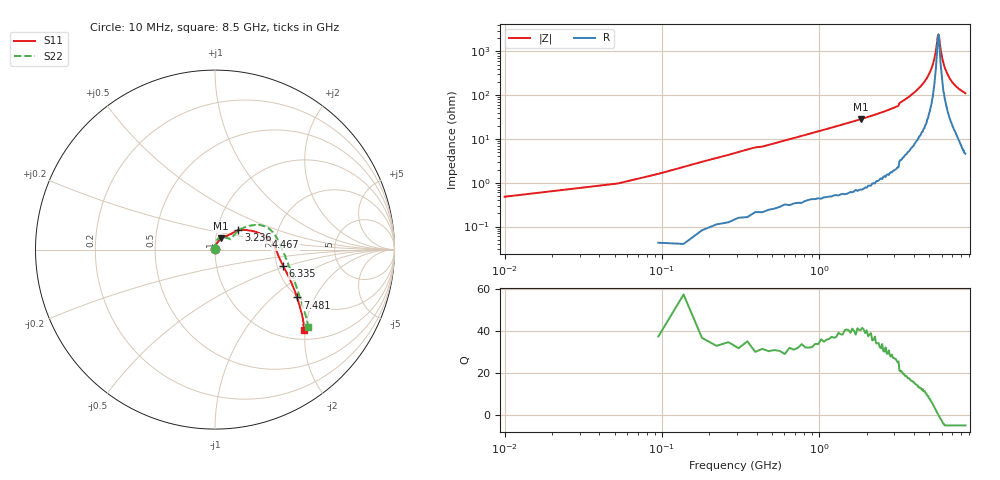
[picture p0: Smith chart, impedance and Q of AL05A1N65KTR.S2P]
!AVX Corporation
!PN: AL05A1N65KTR
!Description: Air Core Inductor, 1.65nH, 2 Turns
!Agilent Technologies,E5071C,MY46102230,A.09.54
!Date: Mon Sep 03 16:13:00 2012
!Data & Calibration Information:
!Freq	S11:SOLT2(ON)	S21:SOLT2(ON)	S12:SOLT2(ON)	S22:SOLT2(ON)
# Hz S dB R 50
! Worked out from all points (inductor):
!   201 points, 10 MHz to 8.5 GHz, reference 50 ohm
!   read as 1/Y11, port 2 shorted: L = 2.67 nH near 52.45 MHz
!   highest Q = 40.6 at 1.835 GHz (marker M1), where L = 2.45 nH
!   self-resonance near 5.728 GHz
!   S11 on the Smith chart (normalised r, x): 10 MHz: 1.00, +0.00; 3.236 GHz: 1.26, +0.28; 4.467 GHz: 1.77, +0.27; 6.335 GHz: 2.16, -0.46; 7.481 GHz: 1.97, -1.46; 8.5 GHz: 1.21, -1.96
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1e7  -58.61 74.1  -0.01 -0.2  -0.10 -0.5  -55.87 62.4
5.245e7  -46.79 83.3  -0.00 -0.8  0.02 -0.9  -46.65 84.5
9.49e7  -42.16 82.5  -0.01 -1.4  0.01 -1.4  -42.47 82.3
1.798e8  -36.85 81.4  -0.01 -2.6  0.00 -2.6  -36.81 82.9
3.496e8  -31.48 78.3  -0.02 -5.0  -0.01 -5.1  -31.54 83.5
3.9205e8  -30.72 78.7  -0.03 -5.6  -0.02 -5.7  -30.74 81.9
4.345e8  -31.84 76.9  -0.03 -6.1  -0.01 -6.2  -31.84 81.7
6.043e8  -29.25 74.1  -0.04 -8.5  -0.03 -8.6  -29.33 79.4
9.0145e8  -26.52 71.2  -0.06 -12.6  -0.05 -12.7  -26.63 77.0
1.4533e9  -24.07 65.9  -0.10 -20.4  -0.10 -20.4  -24.07 72.9
1.83535e9  -22.92 62.6  -0.13 -25.8  -0.13 -25.8  -22.90 67.8
2.85415e9  -20.60 52.3  -0.18 -40.4  -0.18 -40.5  -20.43 42.8
3.19375e9  -19.78 48.6  -0.20 -45.5  -0.19 -45.6  -19.67 33.5
3.2362e9  -15.45 39.9  -0.29 -46.7  -0.29 -46.7  -15.18 40.0
3.70315e9  -13.10 28.6  -0.40 -54.0  -0.40 -54.1  -13.00 35.4
4.255e9  -11.19 17.9  -0.56 -62.9  -0.56 -62.9  -11.21 29.4
4.46725e9  -10.65 13.8  -0.60 -66.4  -0.60 -66.4  -10.62 27.1
5.6983e9  -9.06 -4.5  -0.84 -87.0  -0.84 -87.0  -9.04 9.0
6.33505e9  -8.17 -13.4  -1.06 -98.0  -1.05 -98.0  -8.17 -4.7
7.09915e9  -6.46 -24.8  -1.55 -110.8  -1.55 -110.8  -6.43 -21.6
7.4812e9  -5.52 -30.2  -1.92 -116.3  -1.92 -116.3  -5.44 -28.6
8.5e9  -3.50 -42.3  -3.05 -128.7  -3.05 -128.7  -3.41 -39.8
